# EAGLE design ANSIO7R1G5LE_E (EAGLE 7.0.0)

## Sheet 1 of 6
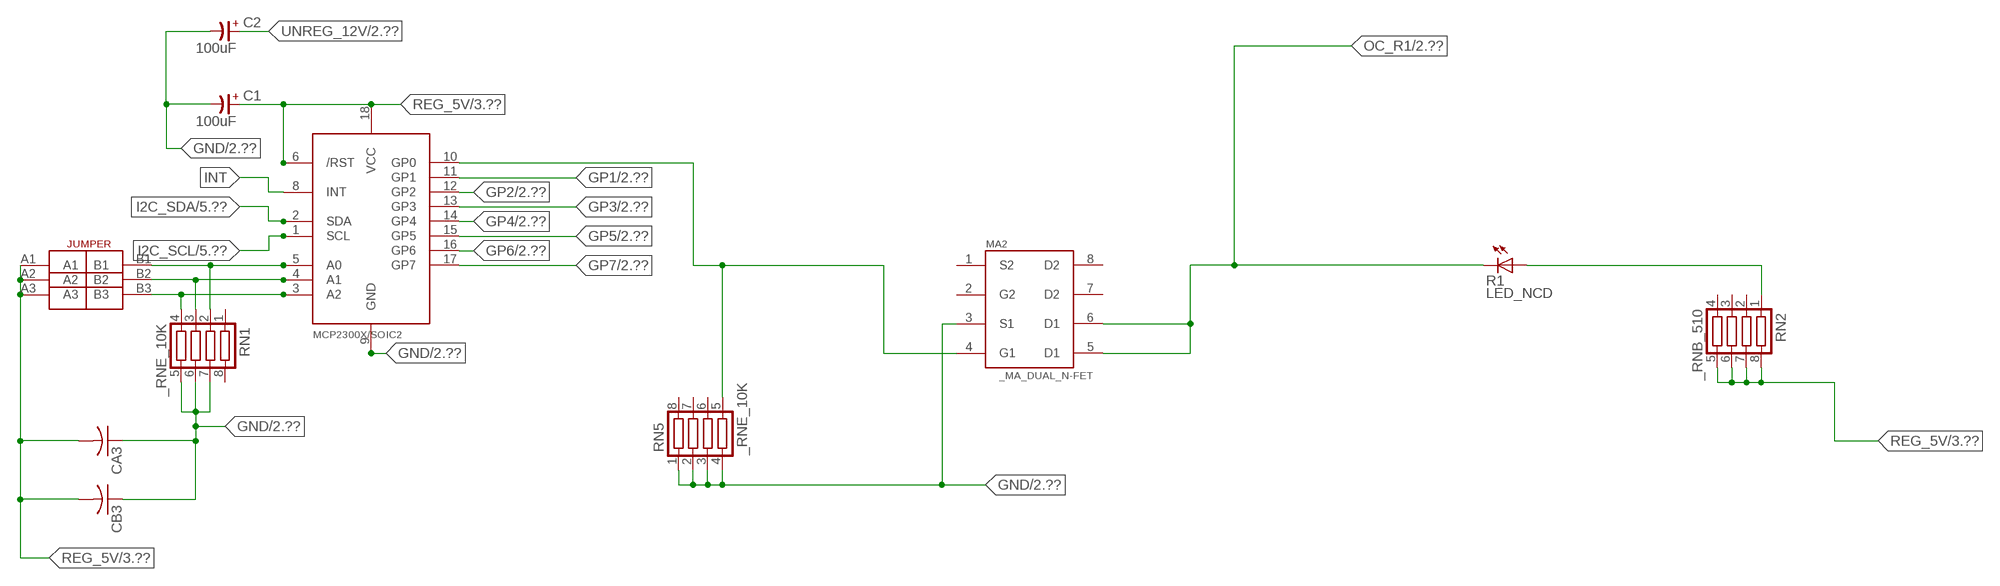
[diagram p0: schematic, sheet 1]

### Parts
C1  100uF  CP-E-025X060  [E-025X060]
C2  100uF  CP-E-025X060  [E-025X060]
CA3  CC1206KRX7R9BB104C1206K  [CC1206KRX7R9BB104]
CB3  TMK316F106ZL-TC1206K  [TMK316F106ZL-T]
IC2  MCP2300X/SO  [SO18W]
MA2  _MA_DUAL_N-FET  [_MA_DUAL_N-FET]
R1  LED_NCD  [CHIPLED_0603]
RN1  _RNE_10K  [RNE]
RN2  _RNB_510  [RNB]
RN5  _RNE_10K  [RNE]
U$18  JUMPER_3X2  [JUMPER_3X2]

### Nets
GND: C1.- C2.- CA3.1 CB3.1 IC2.9(GND) MA2.3(S1) RN1.5 RN1.6 RN1.7 RN5.1 RN5.2 RN5.3 RN5.4 ; also sheet 2,3,4,5,6
GP1: IC2.11(GP1) ; also sheet 2
GP2: IC2.12(GP2) ; also sheet 2
GP3: IC2.13(GP3) ; also sheet 2
GP4: IC2.14(GP4) ; also sheet 2
GP5: IC2.15(GP5) ; also sheet 2
GP6: IC2.16(GP6) ; also sheet 2
GP7: IC2.17(GP7) ; also sheet 2
I2C_SCL: IC2.1(SCL) ; also sheet 5,6
I2C_SDA: IC2.2(SDA) ; also sheet 5,6
INT: IC2.8(INT)
N$6: IC2.5(A0) RN1.2 U$18.B1
N$7: IC2.4(A1) RN1.3 U$18.B2
N$8: IC2.3(A2) RN1.4 U$18.B3
N$23: IC2.10(GP0) MA2.4(G1) RN5.5
N$32: R1.A RN2.1
OC_R1: MA2.5(D1) MA2.6(D1) R1.C ; also sheet 2
REG_5V: C1.+ CA3.2 CB3.2 IC2.6(/RST) IC2.18(VCC) RN2.5 RN2.6 RN2.7 RN2.8 U$18.A1 U$18.A2 U$18.A3 ; also sheet 3,4,5,6
UNREG_12V: C2.+ ; also sheet 2,3
Unconnected: MA2.2(G2) MA2.7(D2) MA2.8(D2) RN1.1 RN1.8 RN2.2 RN2.3 RN2.4 RN5.6 RN5.7 RN5.8

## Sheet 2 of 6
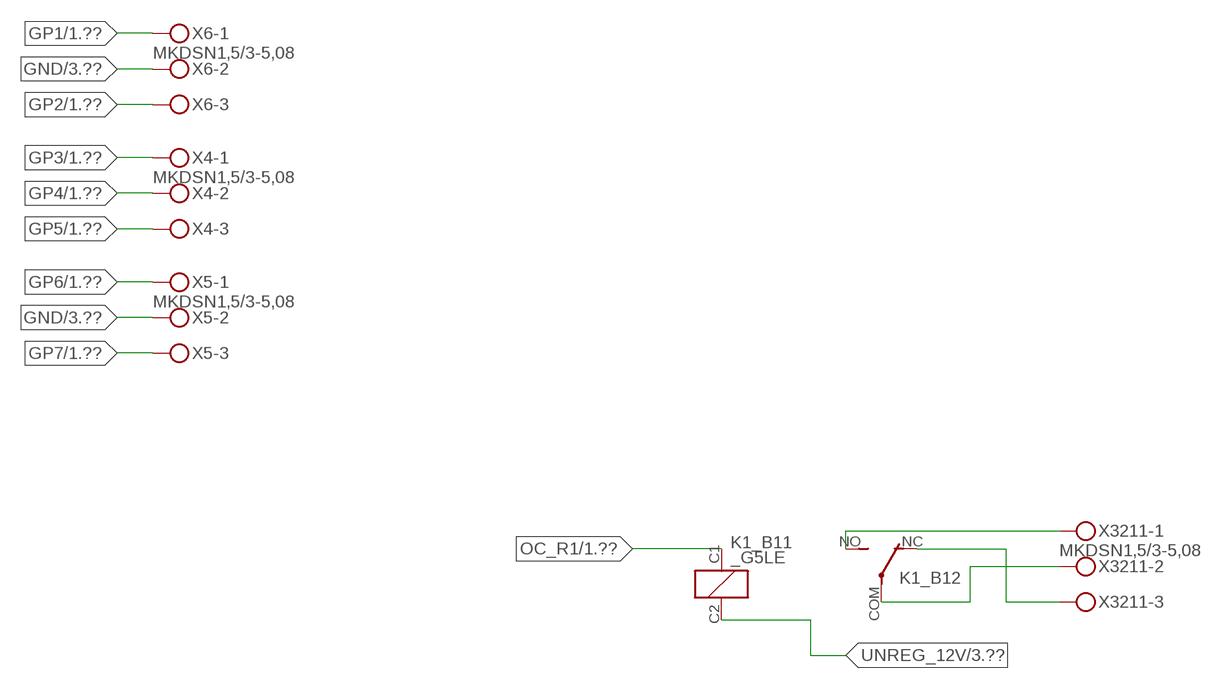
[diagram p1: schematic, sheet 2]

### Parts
K1_B1  _G5LE  [G5LE]
X4  MKDSN1,5/3-5,08  [MKDSN1,5/3-5,08]
X5  MKDSN1,5/3-5,08  [MKDSN1,5/3-5,08]
X6  MKDSN1,5/3-5,08  [MKDSN1,5/3-5,08]
X3211  MKDSN1,5/3-5,08  [MKDSN1,5/3-5,08]

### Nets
GND: X5.2 X6.2 ; also sheet 1,3,4,5,6
GP1: X6.1 ; also sheet 1
GP2: X6.3 ; also sheet 1
GP3: X4.1 ; also sheet 1
GP4: X4.2 ; also sheet 1
GP5: X4.3 ; also sheet 1
GP6: X5.1 ; also sheet 1
GP7: X5.3 ; also sheet 1
N$224: K1_B1.NO(2:NO) X3211.1
N$225: K1_B1.NC(2:NC) X3211.3
N$226: K1_B1.COM(2:COM) X3211.2
OC_R1: K1_B1.C1(1:C1) ; also sheet 1
UNREG_12V: K1_B1.C2(1:C2) ; also sheet 1,3

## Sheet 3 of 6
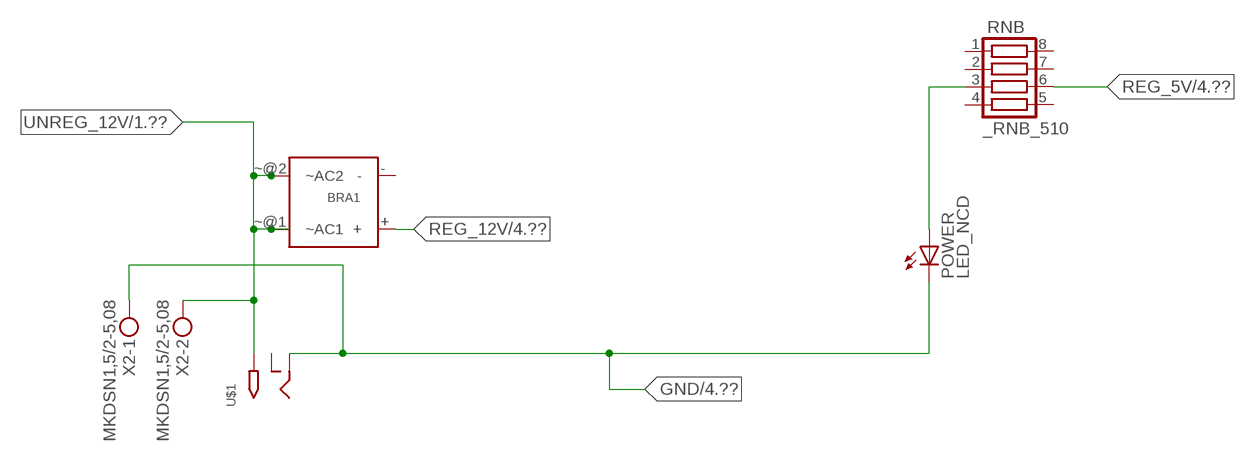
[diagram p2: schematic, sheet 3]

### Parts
BRA1  MB2S_  [MB2S]
POWER  LED_NCD  [CHIPLED_0603]
RNB  _RNB_510  [RNB]
U$1  2.1MMJACK  [PJ-102A]
X2  MKDSN1,5/2-5,08  [MKDSN1,5/2-5,08]

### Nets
GND: POWER.C U$1.RING X2.1 ; also sheet 1,2,4,5,6
N$2: POWER.A RNB.3
REG_5V: RNB.6 ; also sheet 1,4,5,6
REG_12V: BRA1.+ ; also sheet 4
UNREG_12V: BRA1.~@1(~AC1) BRA1.~@2(~AC2) U$1.TIP X2.2 ; also sheet 1,2
Unconnected: BRA1.- RNB.1 RNB.2 RNB.4 RNB.5 RNB.7 RNB.8 U$1.RING_SW

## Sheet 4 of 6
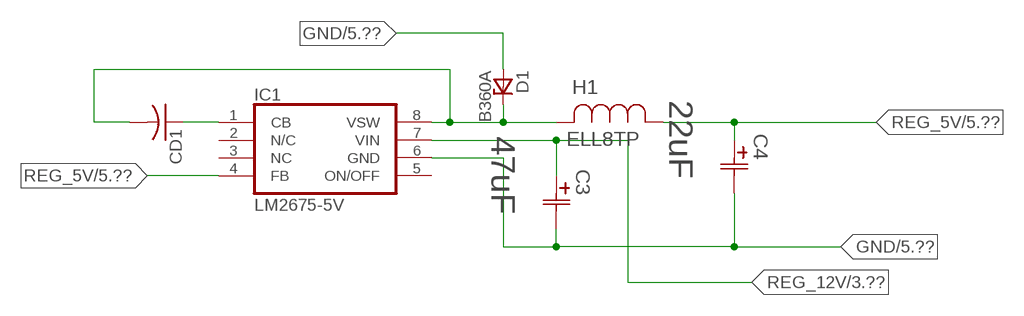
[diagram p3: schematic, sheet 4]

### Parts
C3  47uF  490-5463-6-NDCAP  [C2917(7343)-Y]
C4  22uF  490-5463-6-NDCAP  [C2917(7343)-Y]
CD1  _CD_10NF_50VC1206K  [_CD_10NF_50V]
D1  B360A  [DO214AC_ZENER]
H1  ELL8TP  [IND_ELL8TP]
IC1  LM2675-5V  LM2675  [SO-8]

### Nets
GND: C3.2(C2) C4.2(C2) D1.A IC1.6(GND) ; also sheet 1,2,3,5,6
N$3: CD1.2 D1.C H1.2 IC1.8(VSW)
N$4: CD1.1 IC1.1(CB)
REG_5V: C4.1(C1) H1.1 IC1.4(FB) ; also sheet 1,3,5,6
REG_12V: C3.1(C1) IC1.7(VIN) ; also sheet 3
Unconnected: IC1.2(N/C) IC1.5(ON/OFF)

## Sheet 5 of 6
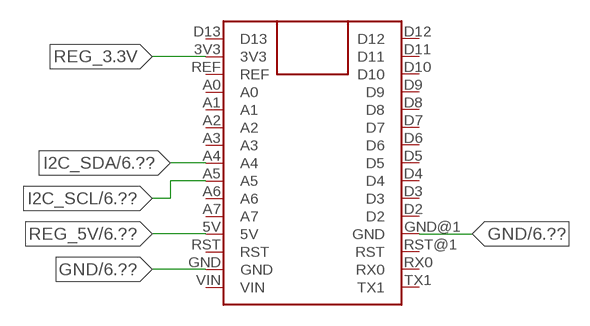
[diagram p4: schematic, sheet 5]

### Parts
FOR_NANO  ARDUINO_NANO  [ARDUINO_NANO]

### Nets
GND: FOR_NANO.GND FOR_NANO.GND@1(GND) ; also sheet 1,2,3,4,6
I2C_SCL: FOR_NANO.A5 ; also sheet 1,6
I2C_SDA: FOR_NANO.A4 ; also sheet 1,6
REG_3.3V: FOR_NANO.3V3
REG_5V: FOR_NANO.5V ; also sheet 1,3,4,6
Unconnected: FOR_NANO.A0 FOR_NANO.A1 FOR_NANO.A2 FOR_NANO.A3 FOR_NANO.A6 FOR_NANO.A7 FOR_NANO.D2 FOR_NANO.D3 FOR_NANO.D4 FOR_NANO.D5 FOR_NANO.D6 FOR_NANO.D7 FOR_NANO.D8 FOR_NANO.D9 FOR_NANO.D10 FOR_NANO.D11 FOR_NANO.D12 FOR_NANO.D13 FOR_NANO.REF FOR_NANO.RST FOR_NANO.RST@1(RST) FOR_NANO.RX0 FOR_NANO.TX1 FOR_NANO.VIN

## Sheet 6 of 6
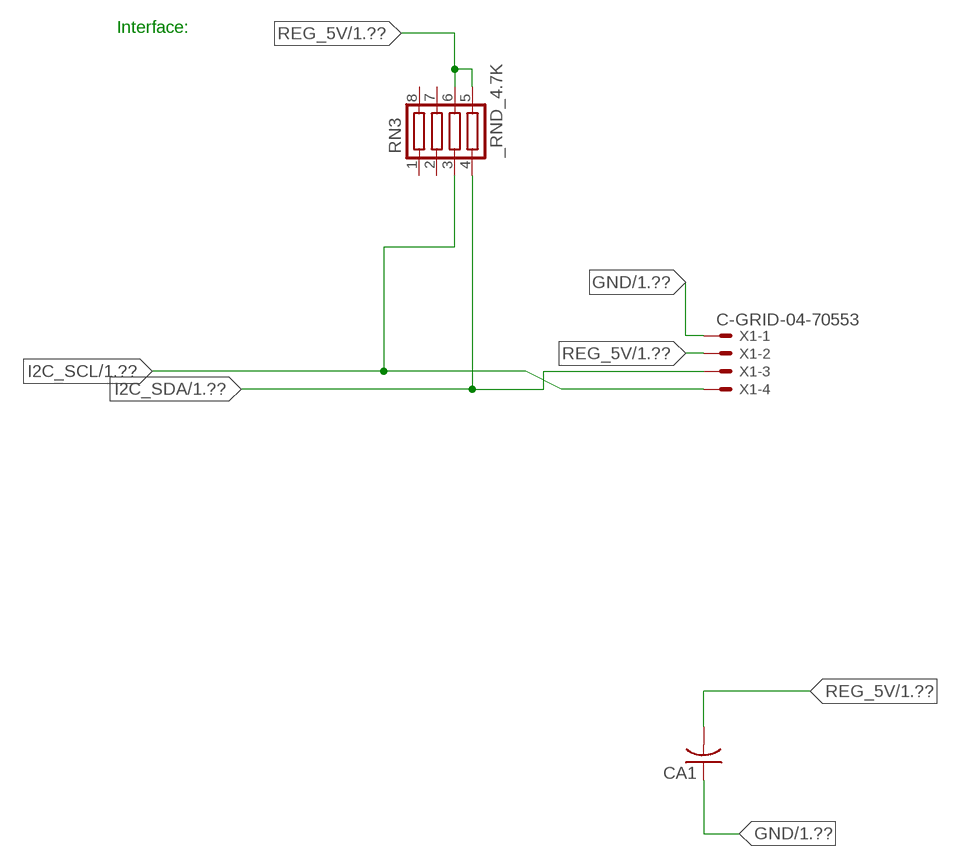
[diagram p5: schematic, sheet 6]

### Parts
CA1  CC1206KRX7R9BB104  [.1UF]
RN3  _RND_4.7K  [RND]
X1  C-GRID-04-70553  [70553-04]

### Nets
GND: CA1.1 X1.1 ; also sheet 1,2,3,4,5
I2C_SCL: RN3.3 X1.4 ; also sheet 1,5
I2C_SDA: RN3.4 X1.3 ; also sheet 1,5
REG_5V: CA1.2 RN3.5 RN3.6 X1.2 ; also sheet 1,3,4,5
Unconnected: RN3.1 RN3.2 RN3.7 RN3.8

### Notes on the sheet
- Interface:

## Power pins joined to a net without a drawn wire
NC: IC1.3(NC)
S2: MA2.1(S2)

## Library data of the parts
BRA1 = NCD_ULTIMATE_LIBRARY:MB2S: Bridge Rectifier BRA MB2S 200V 500ma Digikey MB2S-TPMSTR-ND/MB2S-TP
C1 C2 = NCD_ULTIMATE_LIBRARY:CP-: Capacitors All Kinds POLARIZED CAP
C3 C4 = NCD_ULTIMATE_bhaskar:490-5463-6-ND: NCD CAP
CA1 CA3 = NCD_ULTIMATE_LIBRARY:CC1206KRX7R9BB104: Capacitor CA .1uF 50V SMT C1206K CC1206KRX7R9BB104
CB3 = NCD_ULTIMATE_LIBRARY:TMK316F106ZL-T: Capacitor CB 10uF SMT 1206 TMK316F106ZL-T
CD1 = NCD_ULTIMATE_LIBRARY:_CD_10NF_50V: Capacitor 10nF SMT
D1 = NCD_ULTIMATE_bhaskar:B360A: NCD DIODE B350A/B360A
FOR_NANO = NCD_ULTIMATE_CONNECTORS:ARDUINO_NANO
H1 = NCD_ULTIMATE_bhaskar:ELL8TP: NCD coil
IC1 = NCD_ULTIMATE_bhaskar:LM2675: LM2675 NCD http://www.ti.com/lit/ds/symlink/lm2675.pdf
IC2 = NCD_ULTIMATE_LIBRARY:MCP2300X: Semiconductor Port Expander I/O 8-Bit I2C MCP23008 Inexpensive i2c i/o expander - 8 general purpose i/o pins with optional pullups
K1_B1 = NCD_ULTIMATE_LIBRARY:_G5LE: Relay 5A/10A SPDT; OC_FARNELL: unknown; OC_NEWARK: unknown
MA2 = NCD_ULTIMATE_LIBRARY:_MA_DUAL_N-FET: FET Dual N-Channel 8-SOIC NMOSFET Digikey 785-1064-2-ND/AO4842
POWER = NCD_ULTIMATE_bhaskar:LED_NCD
R1 = NCD_ULTIMATE_LIBRARY:LED_NCD: LED Digikey 754-1132-2-ND/APT2012SRCPRV
RN1 RN5 = NCD_ULTIMATE_LIBRARY:_RNE_10K: Resistor Array RNE SMT 10K x 4 Single Resistor Source: http://www.ctscorp.com/components/Datasheets/CTSChipArrayDs.pdf Digikey 742C083103JPTR-ND/742C083103JP; OC_FARNELL: unknown; OC_NEWARK: unknown
RN2 RNB = NCD_ULTIMATE_LIBRARY:_RNB_510: Resistor Array RNB SMT 510 x 4 Single Resistor Source: http://www.ctscorp.com/components/Datasheets/CTSChipArrayDs.pdf Digikey 742C083511JPTR-ND/ 742C083511JP; OC_FARNELL: unknown; OC_NEWARK: unknown
RN3 = NCD_ULTIMATE_LIBRARY:_RND_4.7K: Resistor Array RND SMT 4.7K x 4 Single Resistor Source: http://www.ctscorp.com/components/Datasheets/CTSChipArrayDs.pdf Digikey 742C083472JPTR-ND/742C083472JP; OC_FARNELL: unknown; OC_NEWARK: unknown
U$1 = NCD_ULTIMATE_CONNECTORS:2.1MMJACK: 2.1mm x 5.5mm DC jack with internal switch. Digikey part #PJ-102A, 4UCON part #05537 By microbuilder.eu
U$18 = NCD_ULTIMATE_CONNECTORS:JUMPER_3X2
X1 = NCD_ULTIMATE_CONNECTORS:C-GRID-04: CONNECTOR 4-Pos I2C wire to board 2.54 mm (0.100") pitch header Digikey WM1342-ND/0015912045; OC_FARNELL: unknown; OC_NEWARK: unknown
X2 = NCD_ULTIMATE_CONNECTORS:MKDSN1,5/2-5,08: MKDSN 1,5/ 2-5,08 Printklemme
X4-X6 X3211 = NCD_ULTIMATE_CONNECTORS:MKDSN1,5/3-5,08: MKDSN 1,5/ 3-5,08 Printklemme Nennstrom: 13,5 A Nennspannung: 250 V Rastermaß: 5,08 mm Polzahl: 3 Anschlussart: Schraubanschluss Montage: Löten Anschlussrichtung Leiter/Platine: 0 ° Artikelnummer: 1729131 Source: http://eshop.phoenixcontact.com .. 1729131.pdf

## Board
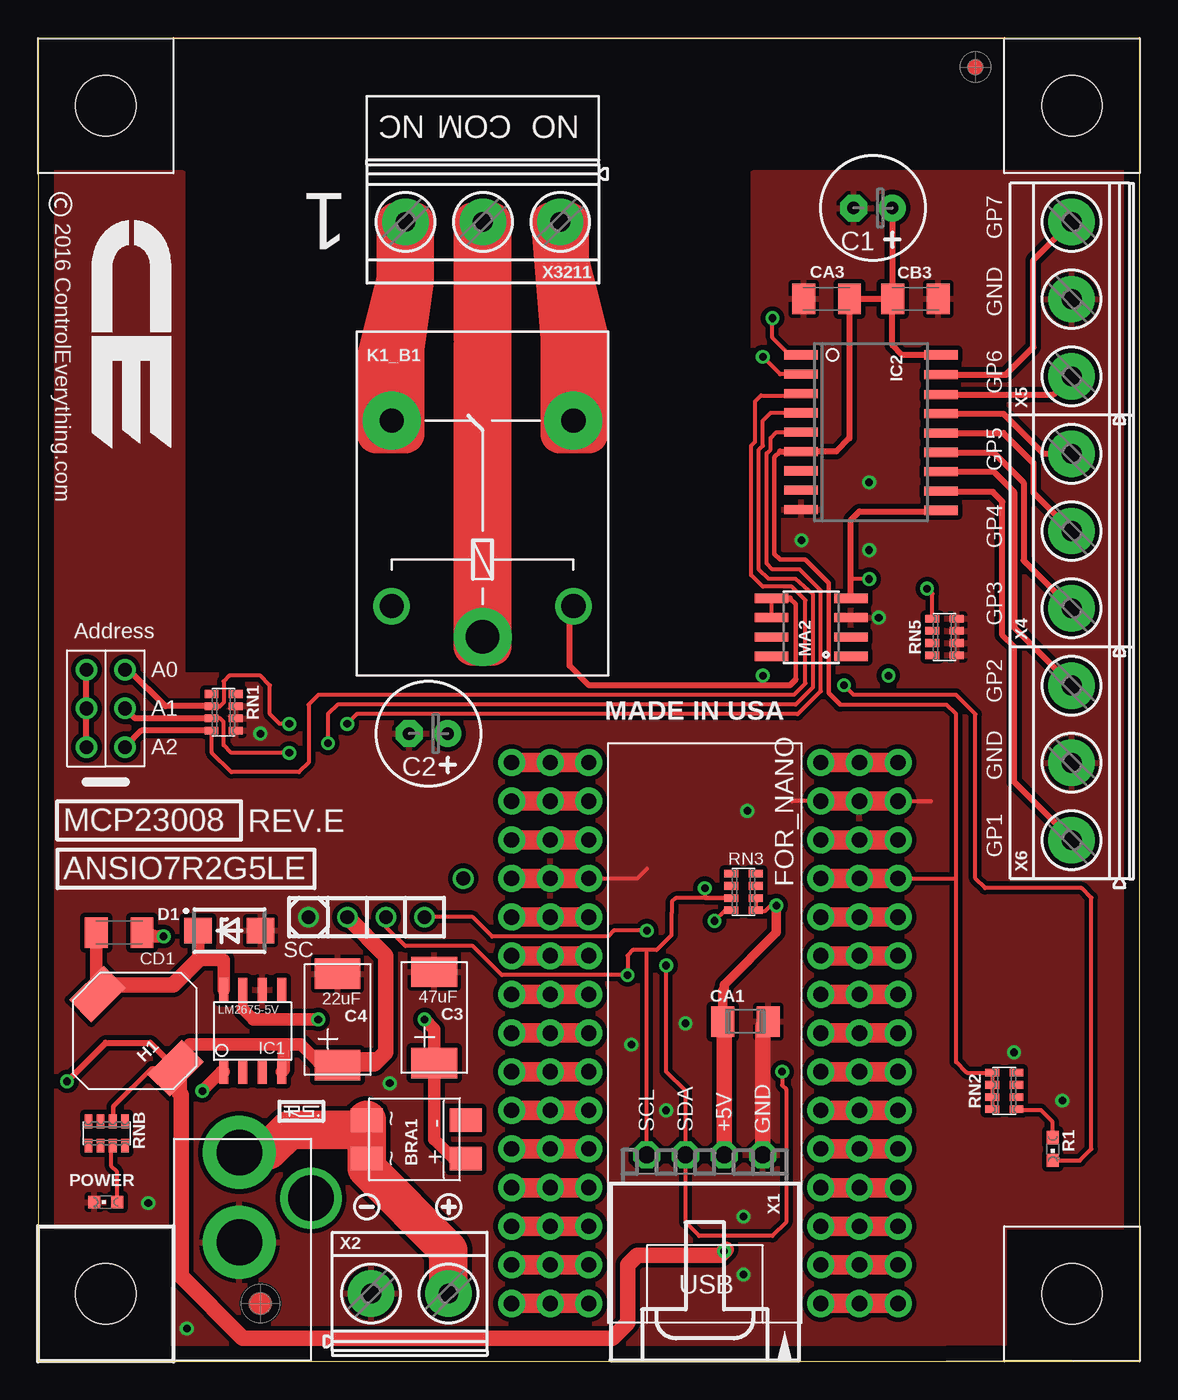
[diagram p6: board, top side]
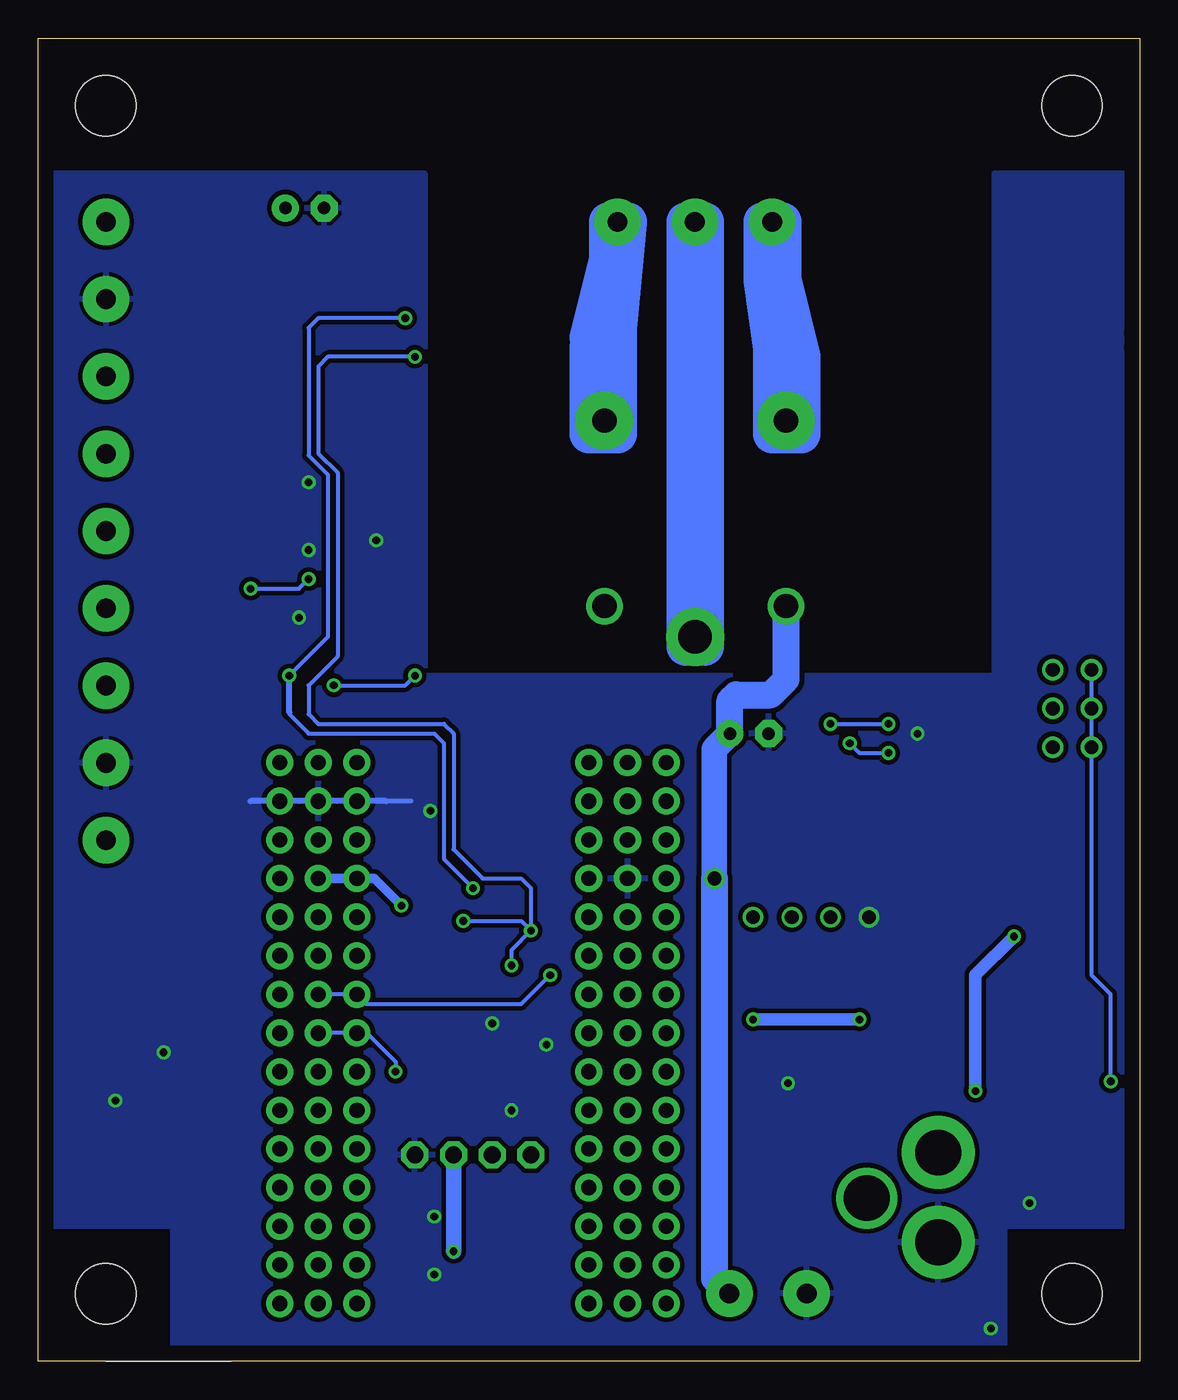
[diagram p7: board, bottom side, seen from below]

Size 72.39 x 87 mm. Coordinates in mm from the lower left corner, seen from the top.
Outline: 0,67.61 0,66.67
Outline: 0,66.67 0,0 59.69,0
Outline: 59.69,0 72.39,0 72.39,87 0,87 0,66.67
Outline: 67.94,0 59.69,0
Copper layers (1*16): Top 0.035mm / dielectric 1.5mm / Bottom 0.035mm
Design rules "default": minimum track width 10mil, minimum drill 24mil, track to track 8mil, track to pad 8mil, pad to pad 8mil, via to via 8mil, smd to smd 8mil, copper to edge 40mil, drill to drill 8mil, minimum pad ring 10mil, minimum via ring 8mil, stop-mask expansion 4mil, vias tented up to drill 0mil, thermal gap 10mil
Holes 3.96 mm at 4.45,4.45 4.45,4.45 4.45,4.45 4.45,4.45

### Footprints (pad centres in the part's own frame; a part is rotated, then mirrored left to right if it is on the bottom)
MB2S = smd 1.55 x 2.1: + 0,-6.5; - 2.54,-6.5; ~@1 0,0; ~@2 2.54,0
E-025X060 = drill 0.813 pad 1.778: + -1.27,0 | drill 0.813 pad 1.778 octagon: - 1.27,0
C2917(7343)-Y = smd 2 x 3: 1 -3,0; 2 3,0
.1UF = smd 1.5 x 2: 1 -1.5,0; 2 1.5,0
CC1206KRX7R9BB104 = smd 1.5 x 2: 1 -1.5,0; 2 1.5,0
TMK316F106ZL-T = smd 1.5 x 2: 1 -1.5,0; 2 1.5,0
_CD_10NF_50V = smd 1.5 x 2: 1 -1.5,0; 2 1.5,0
DO214AC_ZENER = smd 1.8 x 1.7: A 2.05,0; C -2.05,0
ARDUINO_NANO = drill 1 pad 1.778: 3V1 -2.54,-2.54; 3V3 0,-2.54; 5V 0,-27.94; 5V1 -2.54,-27.94; A0 0,-7.62; A1 0,-10.16; A2 0,-12.7; A3 0,-15.24; A4 0,-17.78; A5 0,-20.32; A6 0,-22.86; A7 0,-25.4; A8 -2.54,-7.62; A9 -2.54,-10.16; A10 -2.54,-12.7; A11 -2.54,-15.24; A12 -2.54,-17.78; A13 -2.54,-20.32; A14 -2.54,-22.86; A15 -2.54,-25.4; D1 -2.54,0; D2 20.32,-25.4; D3 20.32,-22.86; D4 20.32,-20.32; D5 20.32,-17.78; D6 20.32,-15.24; D7 20.32,-12.7; D8 20.32,-10.16; D9 20.32,-7.62; D10 20.32,-5.08; D11 20.32,-2.54; D12 20.32,0; D13 0,0; D14 22.86,0; D15 22.86,-2.54; D16 22.86,-5.08; D17 22.86,-7.62; D18 22.86,-10.16; D19 22.86,-12.7; D20 22.86,-15.24; D21 22.86,-17.78; D22 22.86,-20.32; D23 22.86,-22.86; D24 22.86,-25.4; GND 0,-33.02; GND1 -2.54,-33.02; GND@1 20.32,-27.94; GND@2 22.86,-27.94; P$16 2.54,0; P$17 2.54,-2.54; P$18 2.54,-5.08; P$19 2.54,-7.62; P$20 2.54,-10.16; P$21 2.54,-12.7; P$22 2.54,-15.24; P$23 2.54,-17.78; P$24 2.54,-20.32; P$25 2.54,-22.86; P$26 2.54,-25.4; P$27 2.54,-27.94; P$28 2.54,-30.48; P$29 2.54,-33.02; P$30 2.54,-35.56; P$31 17.78,0; P$32 17.78,-2.54; P$33 17.78,-5.08; P$34 17.78,-7.62; P$35 17.78,-10.16; P$36 17.78,-12.7; P$37 17.78,-15.24; P$38 17.78,-17.78; P$39 17.78,-20.32; P$40 17.78,-22.86; P$41 17.78,-25.4; P$42 17.78,-27.94; P$43 17.78,-30.48; P$44 17.78,-33.02; P$45 17.78,-35.56; REF 0,-5.08; REF1 -2.54,-5.08; RST 0,-30.48; RST1 -2.54,-30.48; RST@1 20.32,-30.48; RST@2 22.86,-30.48; RX0 20.32,-33.02; RX1 22.86,-33.02; TX1 20.32,-35.56; TX2 22.86,-35.56; VIN 0,-35.56; VIN1 -2.54,-35.56
IND_ELL8TP = smd 2.054 x 3.2 rotated 45: 1 -2.442,-2.696; 2 2.442,2.442
SO-8 = smd 0.6 x 1.55: 1 -1.905,-2.69; 2 -0.635,-2.69; 3 0.635,-2.69; 4 1.905,-2.69; 5 1.905,2.71; 6 0.635,2.71; 7 -0.635,2.71; 8 -1.905,2.71
SO18W = smd 0.6 x 2.2: 1 -4.445,-4.6; 2 -3.175,-4.6; 3 -1.905,-4.6; 4 -0.635,-4.6; 5 0.635,-4.6; 6 1.905,-4.6; 7 3.175,-4.6; 8 4.445,-4.6; 9 5.715,-4.6; 10 5.775,4.6; 11 4.505,4.6; 12 3.235,4.6; 13 1.965,4.6; 14 0.695,4.6; 15 -0.575,4.6; 16 -1.845,4.6; 17 -3.145,4.6; 18 -4.445,4.6
G5LE = drill 1.6: C1 -7.493,-5.969; C2 -7.493,5.969 | drill 2.2 pad 3.81: COM -9.525,0 | drill 1.6 pad 3.81: NC 4.699,5.969; NO 4.699,-5.969
_MA_DUAL_N-FET = smd 0.61 x 2.21: 1 -1.905,-2.616; 2 -0.635,-2.616; 3 0.635,-2.616; 4 1.905,-2.616; 5 1.905,2.616; 6 0.635,2.616; 7 -0.635,2.616; 8 -1.905,2.616
CHIPLED_0603 = smd 0.8 x 0.8: A 0,-0.75; C 0,0.75
CHIPLED_0603' = smd 0.8 x 0.876: A 0,-0.75; C 0,0.75
RNE = smd 0.5 x 0.9: 1 -1.2,-0.8; 2 -0.4,-0.8; 3 0.4,-0.8; 4 1.2,-0.8; 5 1.2,0.8; 6 0.4,0.8; 7 -0.4,0.8; 8 -1.2,0.8
RNB = smd 0.5 x 0.9: 1 -1.2,-0.8; 2 -0.4,-0.8; 3 0.4,-0.8; 4 1.2,-0.8; 5 1.2,0.8; 6 0.4,0.8; 7 -0.4,0.8; 8 -1.2,0.8
RND = smd 0.5 x 0.9: 1 -1.2,-0.8; 2 -0.4,-0.8; 3 0.4,-0.8; 4 1.2,-0.8; 5 1.2,0.8; 6 0.4,0.8; 7 -0.4,0.8; 8 -1.2,0.8
PJ-102A = drill 3 pad 4.8: RING 0.1,-3.39; TIP 0.1,-9.29 | drill 3 pad 3.251: RING_SW -4.6,-6.29
PCB_MOUNTING_HOLE = hole 3.962: 4.445,4.445
JUMPER_3X2 = drill 0.9: A1 0,5.08; A2 0,2.54; A3 0,0; B1 2.54,5.08; B2 2.54,2.54; B3 2.54,0
70553-04 = drill 1.1 pad 1.778 octagon: 1 -3.81,-7.62; 2 -1.27,-7.62; 3 1.27,-7.62; 4 3.81,-7.62
MKDSN1,5/2-5,08 = drill 1.3 pad 3.048: 1 -2.561,0.025; 2 2.519,0.025
MKDSN1,5/3-5,08 = drill 1.3 pad 3.048: 1 -7.641,0.025; 2 -2.561,0.025; 3 2.519,0.025

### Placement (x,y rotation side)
BRA1  21.59,13.34 90 top
C1  54.86,75.82 180 top
C2  25.65,41.27 180 top
C3  26.04,22.61 90 top
C4  19.68,22.48 90 top
CA1  46.48,22.35 180 top
CA3  51.82,69.85 0 top
CB3  57.66,69.85 180 top
CD1  5.33,28.19 180 top
D1  12.57,28.32 0 top
FOR_NANO  53.98,3.81 180 top
H1  6.35,21.72 90 top
IC1  14.1,21.72 0 top
IC2  54.74,61.72 270 top
K1_B1  29.21,57.15 90 top
MA2  50.8,48.26 90 top
POWER  4.45,10.48 90 top
R1  LED_NCD  [CHIPLED_0603']  66.67,13.97 180 top
RN1  12.19,42.67 270 top
RN2  63.5,17.78 90 top
RN3  46.35,30.86 270 top
RN5  59.56,47.62 90 top
RNB  4.51,14.99 0 top
U$1  13.34,4.45 180 top
U$2  [VISION_REF15]  14.61,3.81 0 top
U$3  [ICON_MINUS]  21.59,10.16 180 top
U$4  PCB_MOUNTING_HOLE  [PCB_MOUNTING_HOLE]  72.39,78.11 90 top
U$5  [ICON_PLUS]  26.99,10.16 90 top
U$6  PCB_MOUNTING_HOLE  [PCB_MOUNTING_HOLE]  72.39,0 90 top
U$11  PCB_MOUNTING_HOLE  [PCB_MOUNTING_HOLE]  8.89,78.11 90 top
U$18  3.17,40.39 0 top
U$19  [VISION_REF10]  61.59,85.09 0 top
U$21  [ICON_USA]  37.21,42.16 0 top
X1  43.81,5.97 180 top
X2  24.45,4.45 0 top
X4  67.94,57.15 90 top
X5  67.94,72.39 90 top
X6  67.94,41.91 90 top
X3211  26.67,74.93 180 top

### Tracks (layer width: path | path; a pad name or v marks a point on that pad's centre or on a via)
GND  (via drill 0.5, 0.9)
  Top 0.254: 36.2,31.75 39.37,31.75 40.01,32.38 | FOR_NANO.GND@1 32.38,31.75 | 49.53,36.83 56.52,36.83 58.67,36.83
  Top 1.016: X1.1 47.62,21.99
  Bottom 0.254: 51.44,36.83 FOR_NANO.GND
  Bottom 0.305: 47.88,36.83 49.53,36.83 51.44,36.83
  Bottom 0.406: 49.53,36.83 58.42,36.83
  other vias: 54.61,53.34 54.61,57.79 64.14,20.32 67.31,17.14 50.16,53.98 55.24,48.9 14.61,41.27 9.78,2.16 17.78,29.21 41.27,16.51 46.35,9.53 46.61,36.2 46.35,5.71 42.55,22.23 38.99,20.83 7.24,10.41 23.11,18.29
  pour Bottom (isolate 0.305): -1.27,8.89 8.89,8.89 8.89,0 63.5,0 63.5,8.89 71.75,8.89 71.75,78.11 46.99,78.11 46.99,45.09 9.53,45.09 9.53,78.11 -1.27,78.11
  pour Top (isolate 0.305): -2.54,8.89 8.89,8.89 8.89,0 63.5,0 63.5,8.89 71.75,8.89 71.75,78.11 46.99,78.11 46.99,45.09 9.53,45.09 9.53,78.11 -2.54,78.11
GP1
  Top 0.406: X6.1 67.92,34.31 64.14,38.1 64.14,46.99 63.37,47.75 63.37,56.52 62.74,57.15 59.4,57.15 IC2.11
GP2
  Top 0.406: IC2.12 62.8,58.49 64.14,57.15 64.14,48.26 67.92,44.48 X6.3
GP3
  Top 0.406: IC2.13 62.8,59.76 64.77,57.79 64.77,52.66 X4.1
GP4
  Top 0.406: IC2.14 63.43,61.03 65.41,59.05 65.41,57.1 X4.2
GP5
  Top 0.406: IC2.15 63.43,62.3 66.04,59.69 67.9,59.69 X4.3
GP6
  Top 0.406: IC2.16 66.74,63.57 X5.1
GP7
  Top 0.406: IC2.17 63.6,64.87 65.41,66.67 65.41,72.39 X5.3
I2C_SCL  (via drill 0.5, 0.9)
  Top 0.254: IC2.1 49.4,66.17 48.26,67.31 v48.26,68.58 | 40.01,27.05 40.64,27.05 41.64,28.05 41.64,29.48 41.66,29.5 41.66,30.23 41.89,30.46 RN3.3 45.54,30.48 43.81,30.48 v43.81,31.12 | 40.01,27.05 39.09,27.05 38.73,26.69 v38.73,25.4 30.48,25.4 28.57,27.3 24.13,27.3 22.86,28.58 v22.86,29.21 | X1.4 40.01,27.05
  Bottom 0.254: v48.26,68.58 53.98,68.58 54.61,67.94 54.61,59.56 53.34,58.29 53.34,47.62 v55.88,45.09 | 55.88,42.67 55.88,42.55 54.61,41.27 46.35,41.27 45.72,40.64 45.72,33.02 v43.81,31.12 | FOR_NANO.A5 51.44,24.13 50.8,23.49 40.64,23.49 v38.73,25.4 38.61,25.53
  Bottom 0.406: 55.88,42.67 v55.88,45.09
I2C_SDA  (via drill 0.5, 0.9)
  Top 0.254: IC2.2 48.77,64.9 v47.62,66.04 | RN3.4 45.16,29.66 v44.45,28.96 | 40,28.33 v40.01,28.32 37.85,28.32 37.47,27.94 29.84,27.94 28.57,29.21 v25.4,29.21 | v41.27,26.04 41.27,19.05 42.55,17.78 X1.3 42.55,9.15 43.44,8.25 48.26,8.25 49.15,9.14 49.15,17.91 48.9,18.16 v48.9,19.05
  Bottom 0.254: v47.62,66.04 53.34,66.04 53.98,65.41 53.98,59.69 52.7,58.42 52.7,46.36 54.61,44.45 54.61,42.55 53.98,41.91 45.72,41.91 45.09,41.27 45.09,33.66 43.18,31.75 40.64,31.75 40.01,31.12 v40.01,28.32 | v44.45,28.96 40.64,28.96 v40.01,28.32 | v41.27,26.04 41.27,27.05 v40.01,28.32 | v48.9,19.05 48.9,19.69 50.8,21.59 FOR_NANO.A4
N$2
  Top 0.254: POWER.A 5.2,12.46 4.83,12.83 4.83,14.1 RNB.3
  Top 0.406: 4.95,14.14 RNB.3
N$3
  Top 0.813: H1.2 3.88,24.77 | D1.C 10.52,26.4 12.19,26.38 IC1.8 | CD1.2 3.83,24.15 4.45,24.77
  Top 1.016: 3.88,24.77 4.45,24.77 8.89,24.77 10.52,26.4
N$4  (via drill 0.5)
  Top 0.813: IC1.1 12.04,19.03 v10.79,17.78 | v8.26,27.94 7.72,27.94 CD1.1
  Bottom 0.813: v10.79,17.78 10.79,25.4 v8.26,27.94
N$6  (via drill 0.5)
  Top 0.254: v20.32,41.91 20.95,42.55 49.91,42.55 51.44,44.07 51.44,50.67 50.04,52.07 48.26,52.07 47.88,52.45 47.88,59.69 48.13,59.94 48.13,60.71 48.51,61.09 IC2.5 50.01,60.96 | v16.51,41.91 15.88,41.91 15.24,42.55 15.24,44.45 14.61,45.09 12.57,45.09 12.19,44.7 12.19,43.31 11.94,43.05 11.41,43.05 RN1.2
  Top 0.406: RN1.2 8.36,43.07 5.97,45.47 U$18.B1
  Bottom 0.254: v20.32,41.91 v16.51,41.91
N$7  (via drill 0.5)
  Top 0.254: v19.05,40.64 19.05,42.55 19.68,43.18 49.78,43.18 50.93,44.32 50.93,50.42 49.78,51.44 48.01,51.44 47.37,52.07 47.37,59.94 47.62,60.2 47.62,61.85 48.13,62.36 IC2.4 50.01,62.23 | v16.51,40.01 12.7,40.01 12.19,40.51 12.19,42.04 11.94,42.29 11.41,42.29 RN1.3
  Top 0.406: RN1.3 6.37,42.27 U$18.B2
  Bottom 0.254: v19.05,40.64 18.41,40.01 v16.51,40.01
N$8
  Top 0.254: RN1.4 11.43,41.43 11.43,40.01 12.7,38.73 17.14,38.73 17.78,39.37 17.78,43.18 18.41,43.82 49.66,43.82 50.42,44.58 50.42,50.04 49.53,50.93 47.62,50.93 46.86,51.69 46.86,60.2 47.12,60.45 47.12,63.12 47.5,63.5 50.01,63.5 IC2.3
  Top 0.406: RN1.4 6.79,41.47 U$18.B3
N$23  (via drill 0.5)
  Top 0.254: RN5.5 58.76,50.46 v58.42,50.8 | v54.61,51.44 53.42,51.44
  Top 0.406: MA2.4 53.42,51.44 53.42,55.32 53.98,55.88 59.27,55.88 IC2.10
  Bottom 0.254: v58.42,50.8 55.24,50.8 v54.61,51.44
N$32
  Top 0.254: R1.A 66.67,15.75 65.91,16.51 64.37,16.51 RN2.1
N$224
  Top 2.54: X3211.1 36.22,67.33 34.92,66.04 34.92,62.1 K1_B1.NO
N$225
  Top 2.54: X3211.3 24.15,71.14 22.86,66.04 22.86,62.23 K1_B1.NC
N$226
  Top 2.54: X3211.2 29.23,70.51 29.21,66.67 K1_B1.COM
N$325
  Top 2.54: 34.31,74.91 34.31,66.06 35.56,66.67 35.56,62.23 35.18,61.85
N$326
  Top 2.54: 24.15,74.91 24.15,71.14 23.5,66.67 23.5,62.1 23.24,61.85
N$327
  Top 2.54: 29.23,74.91 29.23,70.51 29.21,66.67 29.21,47.62
N$328
  Bottom 2.54: 29.21,47.62 29.21,74.88 29.23,74.91
N$329
  Bottom 2.54: 23.24,61.85 23.24,66.42 24.13,71.12 24.13,74.88 24.15,74.91
N$330
  Bottom 2.54: 35.18,61.85 35.18,65.66 36.2,67.31 34.29,74.88 34.31,74.91
N$345
  Top 2.54: 34.29,74.93 34.92,74.93 34.92,69.22 36.2,66.67 36.2,60.96 34.29,60.96 34.29,67.31 | 34.29,67.31 34.29,74.93 | 34.29,74.93 33.66,74.93 34.29,67.31
N$346
  Top 2.54: 29.84,70.48 29.84,74.93 29.21,74.93 | 29.84,70.48 28.57,67.31 | 28.57,67.31 29.84,66.67 | 29.84,66.67 29.84,46.99 28.57,46.99 28.57,66.67 29.21,71.12 29.21,74.93 | 29.21,74.93 28.57,74.93 28.57,67.31 | 29.84,70.48 29.84,66.67
N$347
  Top 2.54: 24.77,74.93 24.77,71.12 24.13,66.67 24.13,60.96 22.23,60.96 22.23,66.04 23.5,71.12 23.5,74.93 24.77,74.93
N$348
  Bottom 2.54: 24.13,74.93 23.5,74.93 23.5,71.12 22.23,66.04 22.23,60.96 24.13,60.96 24.13,66.67 24.77,71.12 24.77,74.93
N$349
  Bottom 2.54: 28.57,74.93 28.57,46.99 29.84,46.99 29.84,74.93 28.57,74.93
N$350
  Bottom 2.54: 33.66,74.93 34.29,67.94 34.29,60.96 36.2,60.96 36.2,66.67 34.92,69.22 34.92,74.93 33.66,74.93
OC_R1  (via drill 0.5)
  Top 0.254: MA2.5 MA2.6 | R1.C 68.47,13.22 69.22,13.97 69.22,30.48 68.58,31.12 62.23,31.12 61.59,31.75 61.59,42.55 60.33,43.82 53.59,43.82 v52.96,44.45 | v47.62,45.09 47.62,44.45
  Top 0.305: 49.4,50.16 49.78,49.78 49.78,44.83
  Top 0.406: MA2.5 49.4,50.16 | 49.78,44.83 49.4,44.45 47.62,44.45 36.2,44.45 34.92,45.72 34.92,49.4 K1_B1.C1
  Bottom 0.254: v52.96,44.45 48.26,44.45 v47.62,45.09
REG_5V  (via drill 0.5, 0.9)
  Top 0.254: RN3.6 RN3.5 47.23,29.59 47.75,29.59 48.13,29.97 v48.51,29.97 | 44.98,24.41 45.09,24.51 | 60.33,31.75 60.33,19.69 61.03,18.98 RN2.5 RN2.6 RN2.7 RN2.8 | 60.33,31.75 60.33,42.55 59.69,43.18 52.7,43.18 | 56.52,31.75 60.33,31.75
  Top 0.305: H1.1 7.46,19.27 4.95,16.76 4.95,15.83 RNB.6 | 48.77,59.82 48.39,59.44 48.39,53.09 48.77,52.7 50.42,52.7 51.94,51.18 51.94,43.94 52.7,43.18
  Top 0.406: v1.91,18.41 4.45,20.95 7.37,20.95 H1.1 | U$18.A3 U$18.A2 U$18.A1 | 48.77,59.82 IC2.6 52.45,59.82 53.32,60.68 CA3.2 CB3.2 56.13,69.83 | IC2.18 56.77,66.17 56.13,66.8 56.13,69.83 | C1.+ 56.13,69.83
  Top 0.61: FOR_NANO.5V 56.52,31.75 | CA1.2 44.98,24.41 | 45.09,24.51 45.09,24.77 48.51,28.19 v48.51,29.97
  Top 0.813: 16.13,20.83 9.96,20.83 H1.1 | 16.13,20.83 17.27,20.83 18.41,19.69 20.75,19.69 C4.1 | IC1.4 16.13,19.15 16.13,20.83
  Top 1.016: H1.1 9.27,18.41 9.27,17.65 9.4,17.53 9.4,5.59 13.46,1.52 37.72,1.52 38.73,2.54 38.73,6.35 39.37,6.98 44.83,6.98 v45.09,7.24 45.21,7.37 | 22.05,19.69 22.23,19.69 22.86,20.32 22.86,26.67 v20.32,29.21 | X1.2 45.09,22.25 CA1.2
  Top 1.27: 20.75,19.69 22.05,19.69
  Bottom 0.254: v1.91,18.41 1.91,24.13 3.17,25.4 U$18.A1
  Bottom 0.61: FOR_NANO.5V 50.29,31.75 v48.51,29.97
  Bottom 1.016: v45.09,7.24 X1.2
REG_12V  (via drill 0.5)
  Top 0.61: IC1.7 13.46,23.16 | 14.1,22.48 14.15,22.48
  Top 0.813: v18.41,22.48 14.15,22.48 13.46,23.16 | v25.4,22.48 26.04,21.84 C3.1 26.04,14.61 27.3,13.34 BRA1.+
  Bottom 0.813: v18.41,22.48 v25.4,22.48
UNREG_12V  (via drill 0.9)
  Top 2.54: X2.2 26.97,7.32 21.59,12.7 BRA1.~@1 21.59,15.24 | 21.59,15.24 BRA1.~@2 | U$1.TIP 15.14,13.87 16.51,15.24 21.59,15.24
  Bottom 1.676: v27.94,31.75 27.94,40.26 C2.+
  Bottom 1.778: K1_B1.C2 23.24,44.83 24.26,43.82 26.54,43.82 26.92,43.43 C2.+ | v27.94,31.75 27.94,5.44 X2.2

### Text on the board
tNames: NC | COM | NO | 1 | 2016 ControlEverything.com | GP7 | GND | GP6 | GP5 | GP4 | GP3 | Address | A0 | GP2 | A1 | A2 | GND | MCP23008 | REV.E | GP1 | ANSIO7R2G5LE | SC | SCL | SDA | +5V | GND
